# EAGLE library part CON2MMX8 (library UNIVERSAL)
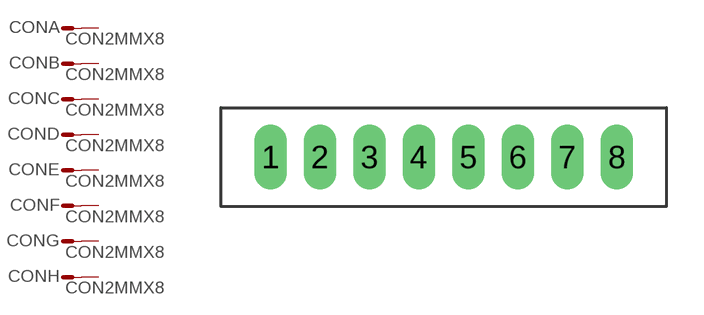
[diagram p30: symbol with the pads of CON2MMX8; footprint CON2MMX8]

Designator prefix CON; gates A=CONPIN B=CONPIN C=CONPIN D=CONPIN E=CONPIN F=CONPIN G=CONPIN H=CONPIN

## CON2MMX8  [CON2MMX8]
1  A:S  pas
2  B:S  pas
3  C:S  pas
4  D:S  pas
5  E:S  pas
6  F:S  pas
7  G:S  pas
8  H:S  pas

## Footprint CON2MMX8 (pad centres in mm)
drill 0.8 pad 1.016 long: 1 2,2; 2 4,2; 3 6,2; 4 8,2; 5 10,2; 6 12,2; 7 14,2; 8 16,2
